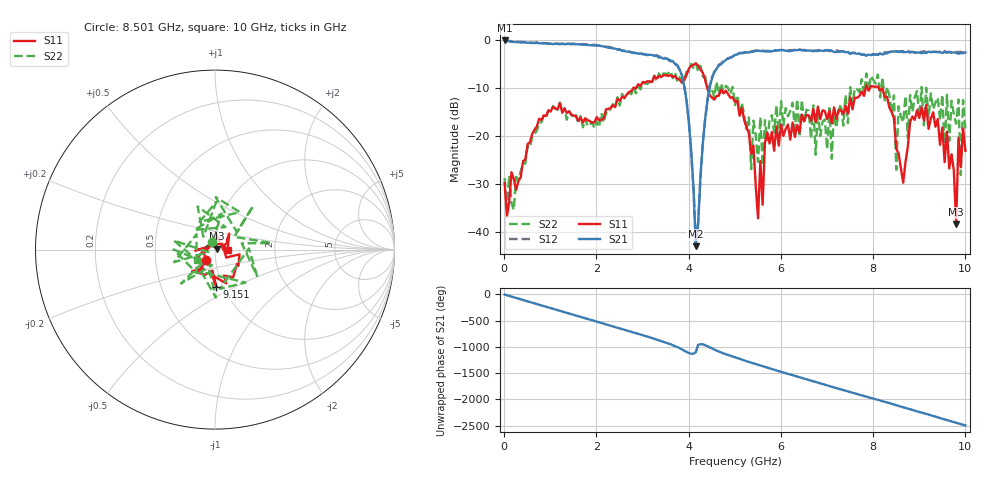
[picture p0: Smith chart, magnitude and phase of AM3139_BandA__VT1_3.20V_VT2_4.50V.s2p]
! Date/Time: Tue, Nov 13, 2018 4:57 PM
! Network Analyzer: Agilent Technologies E8364B Rev: A.07.50.67
! Sweep from 0.010 to 10.000 GHz, 201 Points, Sweep Type: LIN
! Power Supply: 3.201 V, 0.000 A
# Hz S DB R 50
!freq MagS11 AngS11 MagS21 AngS21 MagS12 AngS12 MagS22 AngS22
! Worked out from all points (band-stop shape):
!   201 points, 10 MHz to 10 GHz, reference 50 ohm
!   highest |S21| = -0.18 dB at 10 MHz (marker M1); lowest = -42.9 dB at 4.156 GHz (marker M2)
!   |S21| within 3 dB of the highest: start of sweep to 3.171 GHz; 5.003 GHz to 7.751 GHz (2.749 GHz wide, 43.1 % of centre)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
!   lowest |S11| = -38.4 dB at 9.8 GHz (marker M3), VSWR 1.02, Z = 51.1 + j0.521 ohm
!   |S11| at or under -10 dB: start of sweep to 2.806 GHz; 4.402 GHz to 7.84 GHz (3.439 GHz wide, 56.2 % of centre); 8.118 GHz to end of sweep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
!   |S22| runs from -35.4 to -4.9 dB; largest |S21 - S12| = 0.03
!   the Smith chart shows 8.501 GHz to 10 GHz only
!   S11 on the Smith chart (normalised r, x): 8.501 GHz: 0.90, -0.10; 9.151 GHz: 0.93, -0.41; 10 GHz: 1.15, +0.00
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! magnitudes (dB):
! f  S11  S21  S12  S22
! 10 MHz  -29.8  -0.2  -0.2  -28.8
! 1.708 GHz  -17.2  -1.0  -1.0  -18.2
! 3.357 GHz  -7.6  -3.7  -3.5  -7.0
! 3.906 GHz  -8.4  -9.8  -9.5  -8.3
! 4.156 GHz  -5.0  -42.9  -42.5  -4.9
! 4.456 GHz  -11.6  -10.0  -9.8  -10.8
! 5.005 GHz  -13.0  -3.2  -3.0  -13.6
! 5.505 GHz  -37.2  -2.3  -2.2  -25.4
! 5.704 GHz  -19.3  -2.4  -2.3  -20.9
! 6.703 GHz  -14.4  -2.4  -2.3  -13.7
! 7.103 GHz  -17.4  -2.3  -2.3  -24.8
! 8.352 GHz  -14.1  -2.6  -2.6  -11.6
! 8.501 GHz  -22.7  -2.5  -2.4  -27.1
! 8.551 GHz  -23.7  -2.6  -2.5  -13.8
! 9.151 GHz  -13.6  -2.8  -2.6  -10.0
! 9.55 GHz  -25.5  -2.6  -2.4  -23.0
! 9.6 GHz  -19.1  -2.7  -2.6  -11.5
! 9.8 GHz  -38.4  -2.7  -2.6  -17.5
! 9.85 GHz  -20.4  -3.0  -2.6  -12.4
! 9.9 GHz  -26.5  -2.8  -2.5  -28.1
! 9.95 GHz  -18.4  -2.8  -2.7  -12.6
! 10 GHz  -23.1  -2.7  -2.5  -18.7
